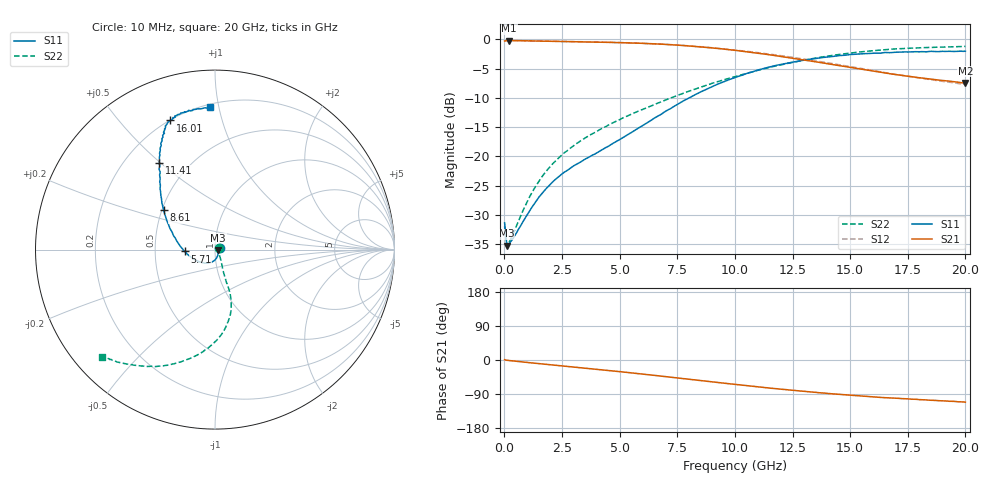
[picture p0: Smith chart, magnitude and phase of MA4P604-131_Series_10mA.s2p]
! AWR Design Environment (9226) Thu Aug 19 15:08:55 2021
! Document = '10mA'
! nPorts: 2, nXvals: 201
# GHz S DB R 50
!Freq DBS11 AngS11 DBS21 AngS21 DBS12 AngS12 DBS22 AngS22
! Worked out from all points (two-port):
!   201 points, 10 MHz to 20 GHz, reference 50 ohm
!   highest |S21| = -0.20 dB at 210 MHz (marker M1); lowest = -7.5 dB at 20 GHz (marker M2)
!   |S21| within 3 dB of the highest: start of sweep to 12.48 GHz
!   lowest |S11| = -35.2 dB at 110 MHz (marker M3), VSWR 1.04, Z = 51.7 - j0.234 ohm
!   |S11| at or under -10 dB: start of sweep to 8.02 GHz
!   |S22| runs from -35.3 to -1.2 dB; largest |S21 - S12| = 0.027
!   S11 on the Smith chart (normalised r, x): 10 MHz: 1.05, +0.01; 5.71 GHz: 0.71, -0.02; 8.61 GHz: 0.51, +0.26; 11.41 GHz: 0.34, +0.50; 16.01 GHz: 0.20, +0.69; 20 GHz: 0.22, +0.94
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0.01  -31.35 13.2  -0.28 0.8  -0.24 0.8  -31.96 26.1
0.11  -35.24 -7.5  -0.21 -0.8  -0.19 -0.7  -35.34 -9.8
0.21  -34.89 -14.7  -0.20 -1.4  -0.19 -1.4  -34.66 -16.4
1.11  -29.23 -63.2  -0.26 -7.2  -0.25 -7.0  -26.79 -53.4
1.61  -26.44 -79.5  -0.30 -10.2  -0.29 -9.9  -23.59 -60.2
2.11  -24.30 -93.6  -0.34 -13.1  -0.32 -12.8  -21.20 -64.8
2.51  -22.97 -104.0  -0.36 -15.5  -0.34 -15.2  -19.69 -67.2
3.41  -20.69 -125.4  -0.42 -21.0  -0.40 -20.4  -17.09 -69.5
4.71  -17.77 -155.4  -0.53 -28.8  -0.52 -28.2  -14.25 -70.7
5.71  -15.41 -176.5  -0.65 -35.3  -0.63 -34.5  -12.43 -70.7
6.71  -13.01 165.8  -0.80 -41.9  -0.79 -41.0  -10.83 -72.1
8.61  -8.81 142.2  -1.32 -54.9  -1.29 -53.6  -8.05 -78.7
10.01  -6.53 130.2  -1.87 -64.5  -1.81 -62.8  -6.37 -86.3
11.41  -4.81 122.8  -2.58 -73.4  -2.48 -71.8  -4.88 -96.4
13.41  -3.31 115.7  -3.78 -84.8  -3.62 -83.7  -3.26 -111.2
14.31  -2.91 113.6  -4.35 -89.3  -4.20 -88.5  -2.69 -117.2
16.01  -2.37 109.1  -5.43 -97.3  -5.35 -96.5  -1.93 -127.0
16.71  -2.28 107.1  -5.86 -100.1  -5.82 -99.3  -1.71 -129.9
18.01  -2.12 102.4  -6.56 -104.6  -6.63 -103.8  -1.43 -133.7
18.21  -2.11 102.5  -6.67 -104.8  -6.74 -104.6  -1.41 -134.5
19.51  -2.07 96.1  -7.23 -109.1  -7.42 -108.5  -1.27 -136.2
20  -2.02 92.2  -7.47 -111.2  -7.70 -110.0  -1.21 -136.6
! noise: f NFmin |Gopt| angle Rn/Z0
0.01  0  1  0  2e-20
2.21  0  1  0  2e-20
4.41  0  1  0  2e-20
6.61  0  1  0  2e-20
8.81  0  1  0  2e-20
11.11  0  1  0  2e-20
13.31  0  1  0  2e-20
15.51  0  1  0  2e-20
17.71  0  1  0  2e-20
20  0  1  0  2e-20
